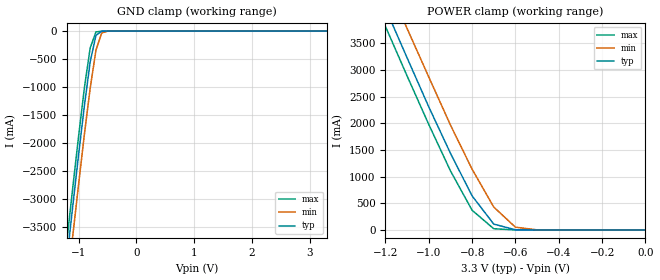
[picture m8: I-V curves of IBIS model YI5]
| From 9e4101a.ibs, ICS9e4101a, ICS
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|   Model YI5
[Model]   YI5
Model_type   Input
Polarity   Inverting
Vinl =   0.35V
Vinh =   0.70V
C_comp   5.50pF   5.00pF   6.00pF
[Temperature Range]   27.00   70.00   0.000
[Voltage Range]   3.30V   3.00V   3.70V
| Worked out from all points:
|   GND clamp passes 1 mA (typ) near -0.54 V on its own axis
|   POWER clamp passes 1 mA (typ) near -0.53 V on its own axis
[GND_clamp]
| voltage   I(typ)   I(min)   I(max)
-3.3V     -24.59A    -25.09A    -24.28A
-1.2V     -4.04A     -4.58A     -3.71A
-1.1V     -3.11A     -3.64A     -2.78A
-1V       -2.2A      -2.73A     -1.87A
-900mV    -1.33A     -1.84A     -1.01A
-800mV    -550mA     -1.02A     -300mA
-700mV    -74.66mA   -340mA     -15.33mA
-600mV    -2.37mA    -33.4mA    -450uA
-500mV    -89.38uA   -1.35mA    -28.49uA
3.3V      71.53pA    2.83uA     48.88pA
[POWER_clamp]
| voltage   I(typ)   I(min)   I(max)
-3.3V     24.72A     25.23A     24.4A
-1.2V     4.16A      4.72A      3.82A
-1.1V     3.23A      3.78A      2.89A
-1V       2.31A      2.87A      1.98A
-900mV    1.44A      1.97A      1.11A
-800mV    640mA      1.14A      370mA
-700mV    110mA      430mA      23.22mA
-600mV    3.5mA      51.94mA    400uA
-500mV    82.64uA    2.18mA     6.3uA
0V        71.53pA    330pA      74.56pA
